(* 	
	Program Name: 	ACS_CMD_START_MOTION
	Purpose:		Copy Start Motion Command to ACS Drive Output Command Register
	When Executed:	Executes current motion command loaded into Output registers
*)
PROGRAM ACS_CMD_START_MOTION
VAR_IN_OUT
	Axis:ACS_DRIVE_TYPE;
END_VAR
VAR
	_command:	USINT	:= ACS_COMMANDS.START_MOTION;
END_VAR

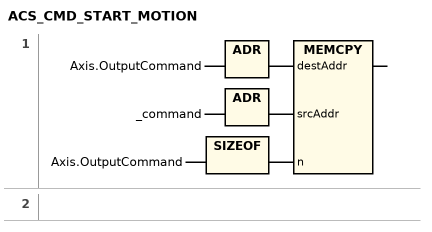
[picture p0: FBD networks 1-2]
// NETWORK 1
MEMCPY(destAddr := ADR(Axis.OutputCommand), srcAddr := ADR(_command), n := SIZEOF(Axis.OutputCommand));

// NETWORK 2

END_PROGRAM
